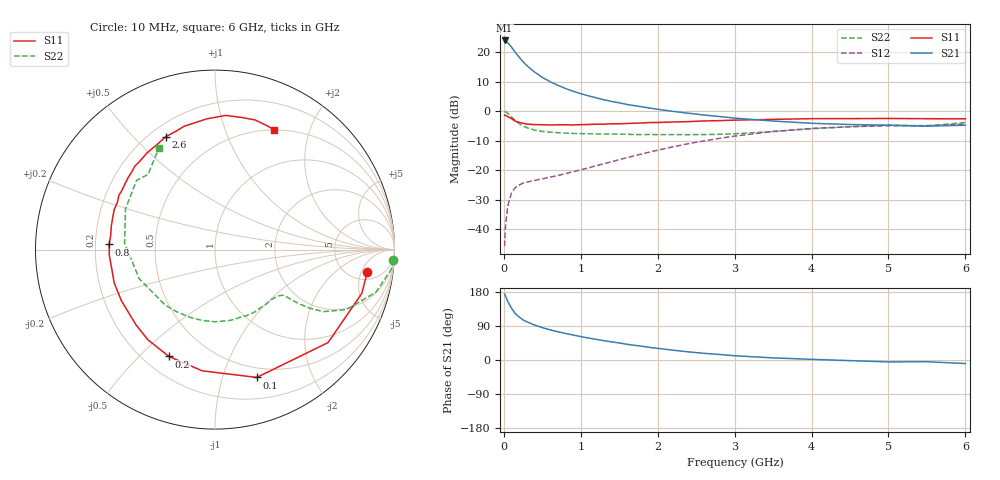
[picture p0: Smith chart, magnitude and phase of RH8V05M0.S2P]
! SIEMENS Small Signal Semiconductors
! BFR106
! Si NPN RF Bipolar Junction Transistor in SOT23
! VCE = 8 V  IC = 5 mA
! Common Emitter S-Parameters:  August  1996
# GHz  S  MA  R  50
!  f  S11  S21  S12  S22
! GHz  MAG  ANG  MAG  ANG  MAG  ANG  MAG  ANG
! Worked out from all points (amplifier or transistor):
!   36 points, 10 MHz to 6 GHz, reference 50 ohm
!   highest |S21| = 24.1 dB at 10 MHz (marker M1)
!   |S21| within 3 dB of that: start of sweep to 119.9 MHz
!   unconditionally stable (mu >= 1): 626.4 MHz to 1.847 GHz; 5.02 GHz to end of sweep
!   at 250 MHz: K = 0.50, MSG = 20.6 dB, |S12| = -24.4 dB
!   at 1.4 GHz: K = 1.13, MAG = 8.1 dB, |S12| = -17.2 dB
!   at 6 GHz: K = 1.02, MAG = -1.0 dB, |S12| = -4.3 dB
!   S11 on the Smith chart (normalised r, x): 10 MHz: 7.00, -6.49; 100 MHz: 0.40, -1.30; 200 MHz: 0.30, -0.62; 800 MHz: 0.26, +0.02; 2.6 GHz: 0.26, +0.62; 6 GHz: 0.50, +1.49
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0.01  0.8579 -8.2  16.02 174.0  0.0051 88.7  0.9948 -3.3
0.02  0.8535 -16.6  15.77 169.7  0.0104 81.4  0.9884 -6.4
0.05  0.8157 -39.4  14.68 154.8  0.0245 69.4  0.9277 -14.8
0.1  0.7493 -71.9  12.33 136.5  0.0412 56.7  0.8041 -24.6
0.15  0.6791 -96.0  9.992 122.3  0.0507 47.4  0.6953 -29.8
0.2  0.6484 -113.3  8.308 113.3  0.056 43.3  0.6184 -31.8
0.25  0.6263 -126.6  6.954 105.8  0.0603 40.5  0.5614 -32.7
0.3  0.6079 -136.4  5.966 100.6  0.0624 40.2  0.5271 -33.1
0.4  0.5942 -151.4  4.654 92.3  0.067 40.6  0.4796 -33.4
0.5  0.5914 -161.7  3.775 85.4  0.0709 42.7  0.4544 -34.0
0.6  0.5851 -170.2  3.196 79.7  0.0761 45.6  0.4427 -35.4
0.8  0.5905 177.2  2.447 70.2  0.0871 51.6  0.4255 -39.4
1.1  0.5972 162.6  1.832 58.0  0.1095 59.4  0.4152 -47.6
1.3  0.604 154.3  1.571 51.0  0.1286 62.8  0.4114 -54.0
1.6  0.6211 143.8  1.308 41.5  0.1627 65.5  0.4074 -64.7
2.2  0.6586 125.0  0.996 25.9  0.2496 63.3  0.402 -90.2
2.6  0.686 113.6  0.865 17.7  0.3136 58.2  0.4022 -110.3
3.5  0.73 93.6  0.683 5.6  0.4552 41.9  0.4525 -159.1
4.5  0.7512 78.4  0.597 -1.7  0.5467 21.5  0.5479 155.5
5  0.756 72.8  0.58 -5.0  0.5681 12.9  0.5828 138.6
5.5  0.7486 67.1  0.56 -4.6  0.5729 8.4  0.561 131.7
6  0.7443 63.7  0.581 -9.3  0.6071 0.2  0.6466 118.9
